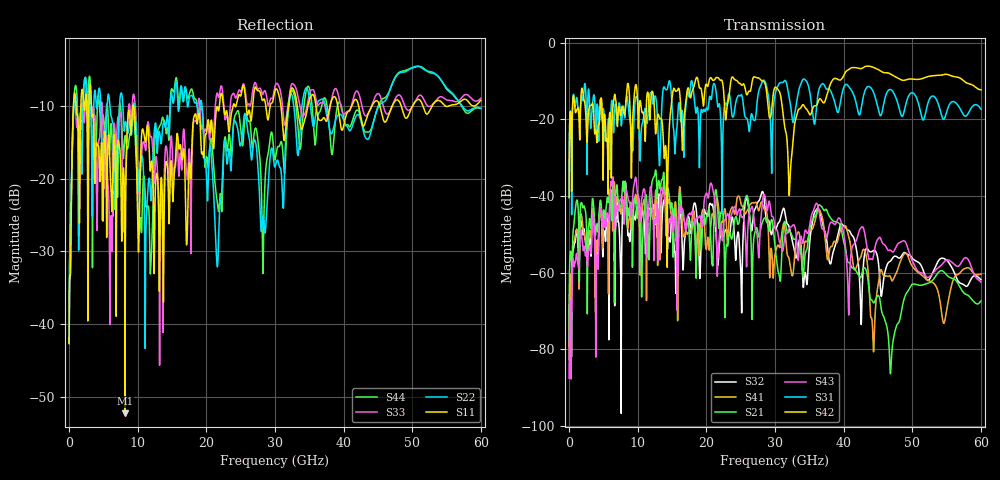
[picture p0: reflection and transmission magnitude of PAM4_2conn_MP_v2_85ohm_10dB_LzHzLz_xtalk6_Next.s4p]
! Info: Touchstone file created by Circ.  Input file=FAB50GbE_2conn_Midplane_Examax_Topo2_v2_85ohm_10dB_LzHzLz.circ
# Hz S RI R 50
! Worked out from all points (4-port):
!   6000 points, 10 MHz to 60 GHz, reference 50 ohm
!   strongest paths, dB at 10 MHz, 15.01 GHz, 30.01 GHz, 45.01 GHz, 60 GHz:
!     S42: -40.3, -14.5, -11.7, -7.0, -12.3
!     S31: -40.5, -16.8, -13.6, -17.1, -17.4
!     S43: -87.5, -45.5, -48.2, -51.2, -62.5
!     S21: -77.6, -42.5, -53.4, -65.9, -67.4
!     S41: -82.6, -46.1, -55.3, -63.5, -60.4
!     S32: -79.1, -44.4, -48.4, -56.6, -61.9
!   lowest |S11| = -52.3 dB at 8.16 GHz (marker M1), VSWR 1.00, Z = 50 + j0.239 ohm
!   |S11| at or under -10 dB: 3.262 GHz to 9.307 GHz (6.045 GHz wide, 96.2 % of centre); 9.409 GHz to 21.9 GHz (12.49 GHz wide, 79.8 % of centre); 35.96 GHz to 38.01 GHz (2.041 GHz wide, 5.52 % of centre)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
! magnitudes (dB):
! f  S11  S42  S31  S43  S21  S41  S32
! 10 MHz  -42.7  -40.3  -40.5  -87.5  -77.6  -82.6  -79.1
! 850 MHz  -8.3  -17.3  -16.5  -57.4  -44.5  -50.8  -52.2
! 8.16 GHz  -52.3  -18.3  -19.1  -41.2  -36.2  -39.5  -37.6
! 21.56 GHz  -10.1  -9.1  -15.2  -58.6  -40.5  -40.6  -54.6
! 36.63 GHz  -12.0  -14.7  -11.3  -46.6  -42.5  -44.2  -45.0
! 46.87 GHz  -10.5  -8.3  -12.3  -54.2  -85.7  -61.3  -56.9
! 60 GHz  -9.2  -12.3  -17.4  -62.5  -67.4  -60.4  -61.9
